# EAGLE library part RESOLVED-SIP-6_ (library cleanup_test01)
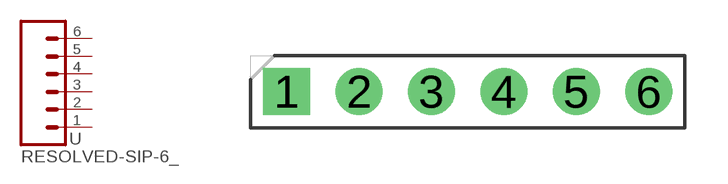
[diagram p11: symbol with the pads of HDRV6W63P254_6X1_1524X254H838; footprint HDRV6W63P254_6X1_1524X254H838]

Designator prefix -

## RESOLVED-SIP-6_2.54-SPACE-VERTICAL  [HDRV6W63P254_6X1_1524X254H838]
1  1  pas
2  2  pas
3  3  pas
4  4  pas
5  5  pas
6  6  pas

## Footprint HDRV6W63P254_6X1_1524X254H838 (pad centres in mm)
drill 1.1 pad 1.65 square: 1 0,0
drill 1.1 pad 1.65: 2 2.54,0; 3 5.08,0; 4 7.62,0; 5 10.16,0; 6 12.7,0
